(* Logix 5000 AddOnInstructionDefinition export SPEL_BaseSet; software revision 30.01 *)

ADD_ON_INSTRUCTION SPEL_ExecCmd   (* revision 1.2 *)
// Executes a command in the robot controller.  Normally this is called by higher level AOIs.
VAR_INPUT
   Start : BOOL; {required}
   MaxTime : DINT := 3000; {required}
END_VAR
VAR_OUTPUT
   InCycle : BOOL; {access Read Only, visible}
   Done : BOOL; {access Read Only, visible}
   Error : BOOL; {access Read Only, visible}
END_VAR
VAR_IN_OUT
   ExtInputs : AB:ETHERNET_MODULE_INT_128Bytes:I:0; {required}
        .DATA[0].0   // ExtCmdGet
        .DATA[0].1   // ExtRespSet
        .DATA[0].2   // ExtCmdResult
        .DATA[0].3   // ExtError
   ExtOutputs : AB:ETHERNET_MODULE_INT_128Bytes:O:0; {required}
        .DATA[0].0   // ExtCmdSet
        .DATA[0].1   // ExtRespGet
        .DATA[0].2   // ExtCmdReset
END_VAR
VAR_INPUT
   Cmd : INT; {required}
   CmdParam1 : INT; {required}
   CmdParam2 : INT; {required}
   CmdParam3 : INT; {required}
   CmdParam4 : INT; {required}
   CmdParam5 : INT; {required}
   CmdParam6 : INT; {required}
   CmdParam7 : INT; {required}
END_VAR
VAR_OUTPUT
   CmdEcho : INT; {access Read Only, visible}
   Resp1 : INT; {access Read Only, visible}
   Resp2 : INT; {access Read Only, visible}
   Resp3 : INT; {access Read Only, visible}
   Resp4 : INT; {access Read Only, visible}
   Resp5 : INT; {access Read Only, visible}
   Resp6 : INT; {access Read Only, visible}
   Resp7 : INT; {access Read Only, visible}
   ErrCode1 : INT; {access Read Only, visible}
   ErrCode2 : INT; {access Read Only, visible}
END_VAR
VAR
   ExtReset : BOOL; {access None}
   ExtError : BOOL; {access None}
   ExtCmdSet : BOOL; {access None}   // Cmd Ready
   ExtCmdGet : BOOL; {access None}   // Cmd Received
   CmdXferDone : BOOL; {access None}
   ExtRespSet : BOOL; {access None}   // Resp Ready
   RespXferDone : BOOL; {access None}
   ExtCmdResult : BOOL; {access None}   // Normal or Error?
   TmrCmdDataRdy : TIMER := (PRE := 5); {access None}
   OneShotDoneOff : BOOL; {access None}
   OneShotStart : BOOL; {access None}
   StartInit : BOOL; {access None}
   OneShotStartError : BOOL; {access None}
   TmrCycle : TIMER := (PRE := 5000); {access None}
   OneshotTmrPreset : BOOL; {access None}
   TmrCmdSet : TIMER := (PRE := 20); {access None}
   OnShotCmdDataXfer : BOOL; {access None}
   OneShotRespDataXfer : BOOL; {access None}
   OneShotDataRdy : BOOL; {access None}
   OtherCmdInCycle : BOOL; {access None}
   s : BOOL; {access None}
   OneShotUnsetCmdIncycle : BOOL; {access None}
   OneShotSetCmdIncycle : BOOL; {access None}
   OneShotSetOtherCmdInCycleError : BOOL; {access None}
   OneShotSetBit : BOOL; {access None}
   MaxTimeError : BOOL; {access None}
END_VAR

ROUTINE Logic   (* ladder *)
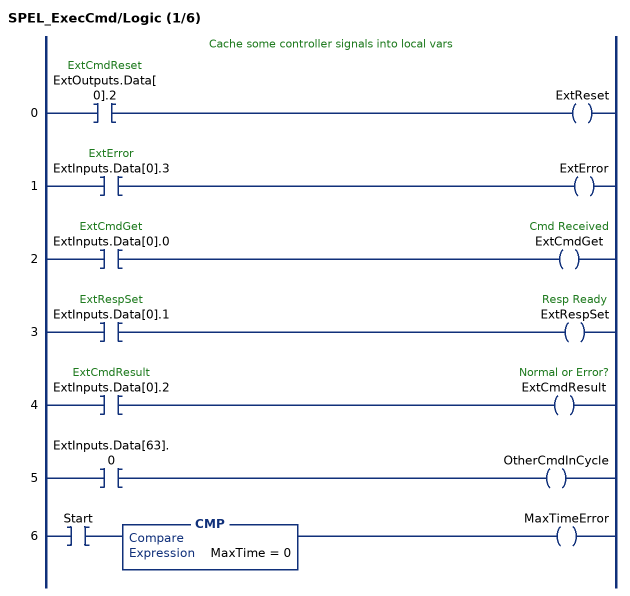
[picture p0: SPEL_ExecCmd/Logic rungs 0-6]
   // Cache some controller signals into local vars
   0: XIC(ExtOutputs.Data[0].2)OTE(ExtReset);
   1: XIC(ExtInputs.Data[0].3)OTE(ExtError);
   2: XIC(ExtInputs.Data[0].0)OTE(ExtCmdGet);
   3: XIC(ExtInputs.Data[0].1)OTE(ExtRespSet);
   4: XIC(ExtInputs.Data[0].2)OTE(ExtCmdResult);
   5: XIC(ExtInputs.Data[63].0)OTE(OtherCmdInCycle);
   6: XIC(Start)CMP(MaxTime = 0)OTE(MaxTimeError);
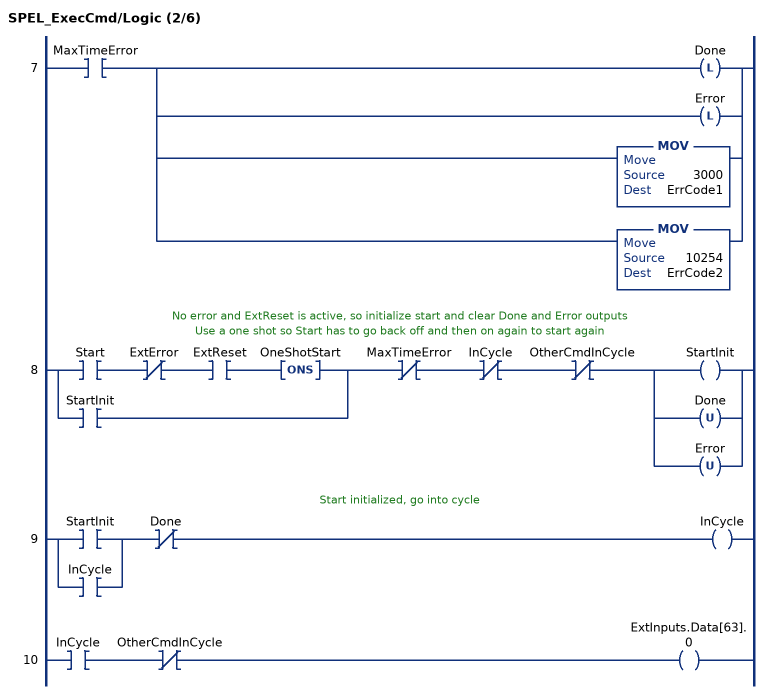
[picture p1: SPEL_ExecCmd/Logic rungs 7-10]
   7: XIC(MaxTimeError)[OTL(Done) ,OTL(Error) ,MOV(3000,ErrCode1) ,MOV(10254,ErrCode2) ];
   // No error and ExtReset is active, so initialize start and clear Done and Error outputs
   // Use a one shot so Start has to go back off and then on again to start again
   8: [XIC(Start) XIO(ExtError) XIC(ExtReset) ONS(OneShotStart) ,XIC(StartInit) ]XIO(MaxTimeError)XIO(InCycle)XIO(OtherCmdInCycle)[OTE(StartInit) ,OTU(Done) ,OTU(Error) ];
   // Start initialized, go into cycle
   9: [XIC(StartInit) ,XIC(InCycle) ]XIO(Done)OTE(InCycle);
   10: XIC(InCycle)XIO(OtherCmdInCycle)OTE(ExtInputs.Data[63].0);
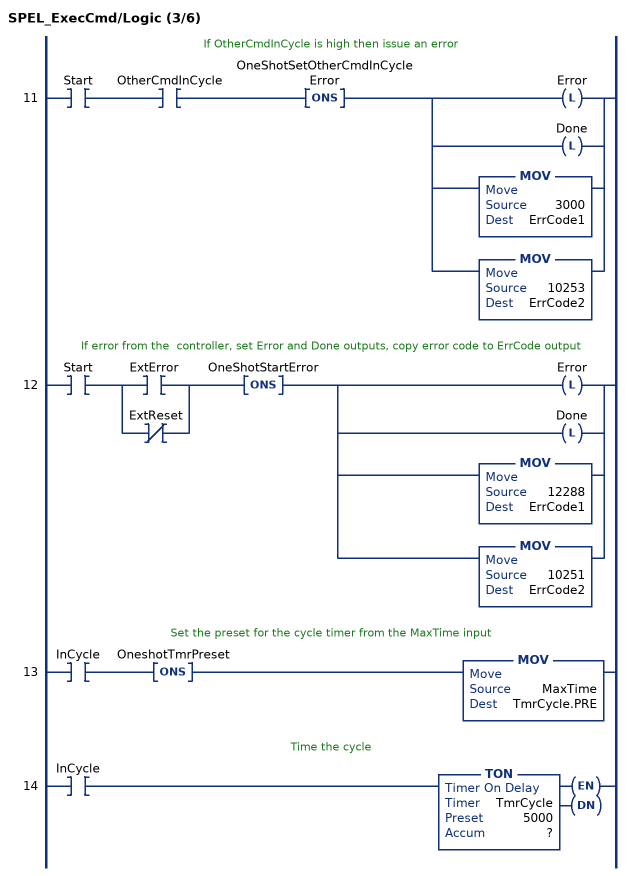
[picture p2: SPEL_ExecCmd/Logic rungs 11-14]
   // If OtherCmdInCycle is high then issue an error
   11: XIC(Start)XIC(OtherCmdInCycle)ONS(OneShotSetOtherCmdInCycleError)[OTL(Error) ,OTL(Done) ,MOV(3000,ErrCode1) ,MOV(10253,ErrCode2) ];
   // If error from the  controller, set Error and Done outputs, copy error code to ErrCode output
   12: XIC(Start)[XIC(ExtError) ,XIO(ExtReset) ]ONS(OneShotStartError)[OTL(Error) ,OTL(Done) ,MOV(12288,ErrCode1) ,MOV(10251,ErrCode2) ];
   // Set the preset for the cycle timer from the MaxTime input
   13: XIC(InCycle)ONS(OneshotTmrPreset)MOV(MaxTime,TmrCycle.PRE);
   // Time the cycle
   14: XIC(InCycle)TON(TmrCycle,?,?);
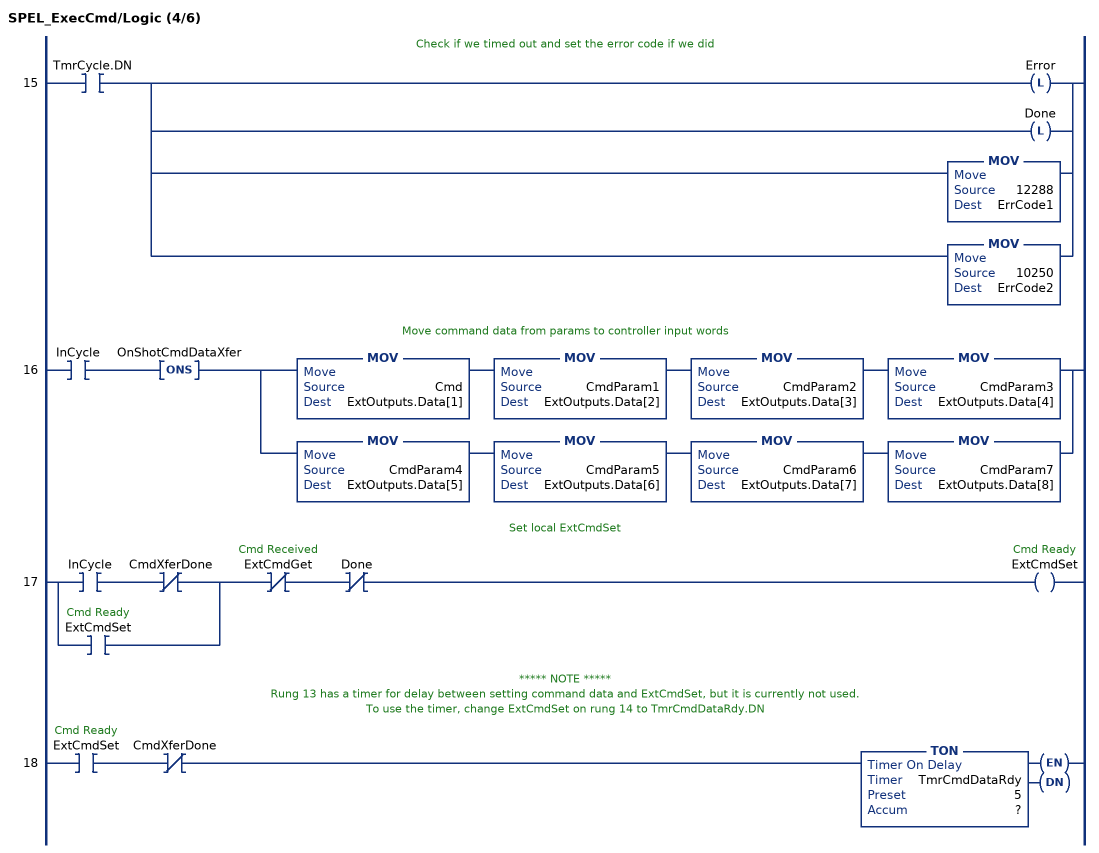
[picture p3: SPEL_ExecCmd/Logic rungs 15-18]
   // Check if we timed out and set the error code if we did
   15: XIC(TmrCycle.DN)[OTL(Error) ,OTL(Done) ,MOV(12288,ErrCode1) ,MOV(10250,ErrCode2) ];
   // Move command data from params to controller input words
   16: XIC(InCycle)ONS(OnShotCmdDataXfer)[MOV(Cmd,ExtOutputs.Data[1]) MOV(CmdParam1,ExtOutputs.Data[2]) MOV(CmdParam2,ExtOutputs.Data[3]) MOV(CmdParam3,ExtOutputs.Data[4]) ,MOV(CmdParam4,ExtOutputs.Data[5]) MOV(CmdParam5,ExtOutputs.Data[6]) MOV(CmdParam6,ExtOutputs.Data[7]) MOV(CmdParam7,ExtOutputs.Data[8]) ];
   // Set local ExtCmdSet
   17: [XIC(InCycle) XIO(CmdXferDone) ,XIC(ExtCmdSet) ]XIO(ExtCmdGet)XIO(Done)OTE(ExtCmdSet);
   // ***** NOTE *****
   // Rung 13 has a timer for delay between setting command data and ExtCmdSet, but it is currently not used.
   // To use the timer, change ExtCmdSet on rung 14 to TmrCmdDataRdy.DN
   18: XIC(ExtCmdSet)XIO(CmdXferDone)TON(TmrCmdDataRdy,?,?);
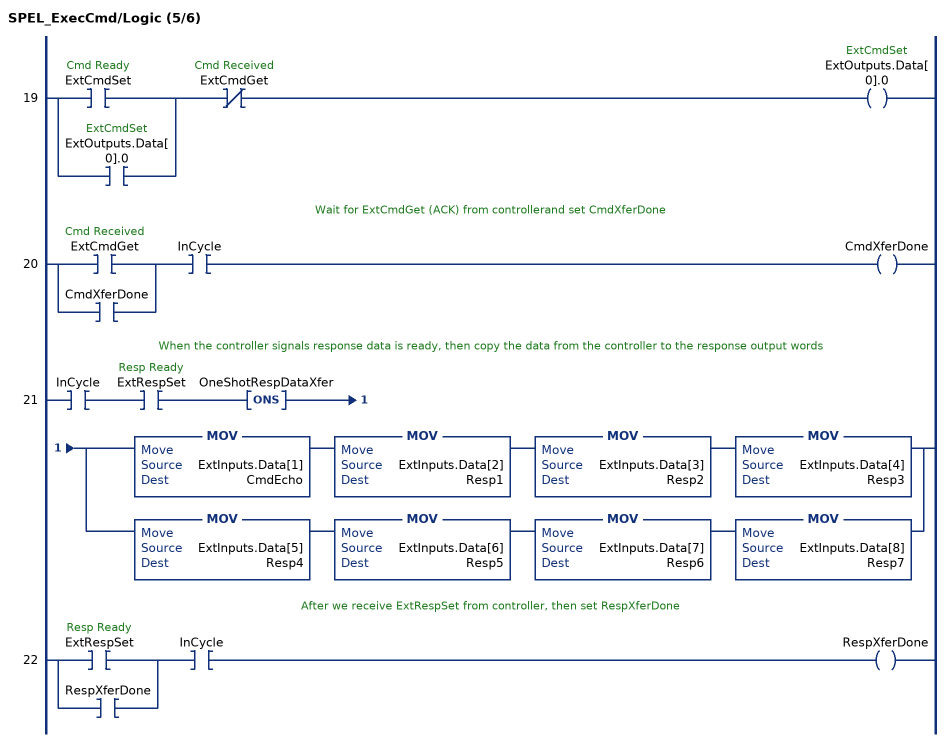
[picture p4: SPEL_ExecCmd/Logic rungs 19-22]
   19: [XIC(ExtCmdSet) ,XIC(ExtOutputs.Data[0].0) ]XIO(ExtCmdGet)OTE(ExtOutputs.Data[0].0);
   // Wait for ExtCmdGet (ACK) from controllerand set CmdXferDone
   20: [XIC(ExtCmdGet) ,XIC(CmdXferDone) ]XIC(InCycle)OTE(CmdXferDone);
   // When the controller signals response data is ready, then copy the data from the controller to the response output words
   21: XIC(InCycle)XIC(ExtRespSet)ONS(OneShotRespDataXfer)[MOV(ExtInputs.Data[1],CmdEcho) MOV(ExtInputs.Data[2],Resp1) MOV(ExtInputs.Data[3],Resp2) MOV(ExtInputs.Data[4],Resp3) ,MOV(ExtInputs.Data[5],Resp4) MOV(ExtInputs.Data[6],Resp5) MOV(ExtInputs.Data[7],Resp6) MOV(ExtInputs.Data[8],Resp7) ];
   // After we receive ExtRespSet from controller, then set RespXferDone
   22: [XIC(ExtRespSet) ,XIC(RespXferDone) ]XIC(InCycle)OTE(RespXferDone);
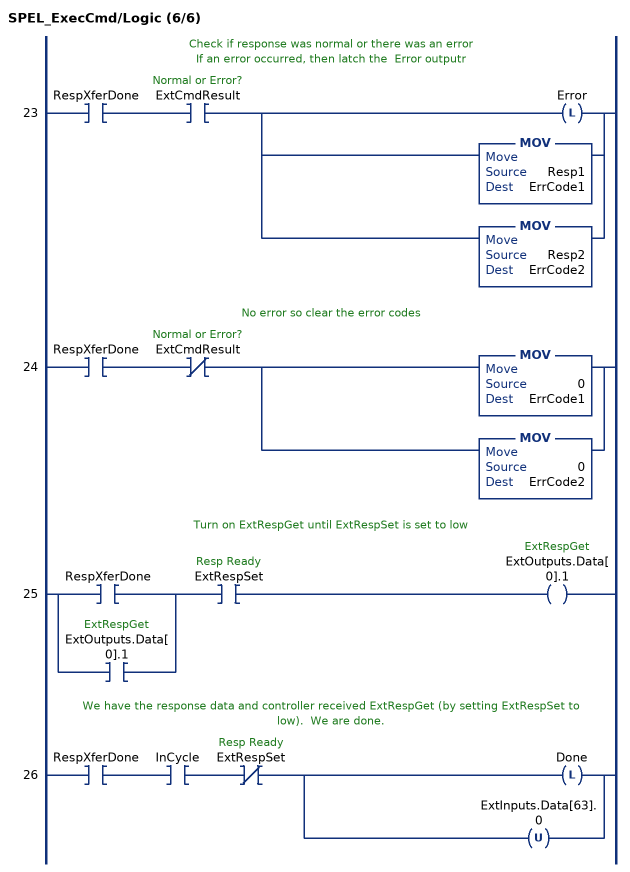
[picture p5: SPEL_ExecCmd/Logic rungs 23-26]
   // Check if response was normal or there was an error
   // If an error occurred, then latch the  Error outputr
   23: XIC(RespXferDone)XIC(ExtCmdResult)[OTL(Error) ,MOV(Resp1,ErrCode1) ,MOV(Resp2,ErrCode2) ];
   // No error so clear the error codes
   24: XIC(RespXferDone)XIO(ExtCmdResult)[MOV(0,ErrCode1) ,MOV(0,ErrCode2) ];
   // Turn on ExtRespGet until ExtRespSet is set to low
   25: [XIC(RespXferDone) ,XIC(ExtOutputs.Data[0].1) ]XIC(ExtRespSet)OTE(ExtOutputs.Data[0].1);
   // We have the response data and controller received ExtRespGet (by setting ExtRespSet to low).  We are done.
   26: XIC(RespXferDone)XIC(InCycle)XIO(ExtRespSet)[OTL(Done) ,OTU(ExtInputs.Data[63].0) ];
END_ROUTINE
END_ADD_ON_INSTRUCTION

ADD_ON_INSTRUCTION SPEL_BaseSet   (* revision 1.2, vendor SEIKO EPSON CORP. *)
// Sets the base coordinate system.
VAR_OUTPUT
   InCycle : BOOL; {access Read Only, visible}
   Done : BOOL; {access Read Only, visible}
END_VAR
VAR_INPUT
   Start : BOOL; {required}
END_VAR
VAR_OUTPUT
   Error : BOOL; {access Read Only, visible}
END_VAR
VAR_INPUT
   NumAxes : INT; {required}
   BaseX : REAL; {required}
   BaseY : REAL; {required}
   BaseZ : REAL; {required}
   BaseU : REAL; {required}
   BaseV : REAL; {required}
   BaseW : REAL; {required}
END_VAR
VAR_IN_OUT
   ExtInputs : AB:ETHERNET_MODULE_INT_128Bytes:I:0; {required}
   ExtOutputs : AB:ETHERNET_MODULE_INT_128Bytes:O:0; {required}
END_VAR
VAR_OUTPUT
   ErrCode1 : INT; {access Read Only, visible}
   ErrCode2 : INT; {access Read Only, visible}
END_VAR
VAR
   Valuex1000 : DINT; {access None}
   Value_INTS : INT[2]; {access None}
   StartInit : BOOL[32]; {access None}
   OneShotStart : BOOL[32]; {access None}
   ExecBaseSetX : SPEL_ExecCmd := (MaxTime := 3000); {access None}
   ExecBaseSetW : SPEL_ExecCmd := (MaxTime := 3000); {access None}
   ExecBaseSetV : SPEL_ExecCmd := (MaxTime := 3000); {access None}
   ExecBaseSetU : SPEL_ExecCmd := (MaxTime := 3000); {access None}
   ExecBaseSetZ : SPEL_ExecCmd := (MaxTime := 3000); {access None}
   ExecBaseSetY : SPEL_ExecCmd := (MaxTime := 3000); {access None}
   X6 : BOOL; {access None}
   ExecTimeout : DINT; {access None}
END_VAR

ROUTINE Logic   (* ladder *)
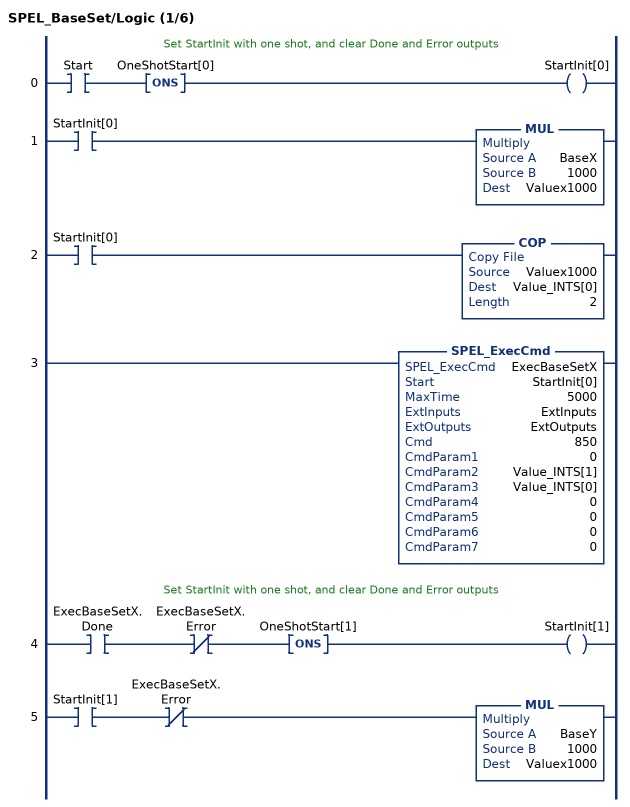
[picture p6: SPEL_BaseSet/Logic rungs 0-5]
   // Set StartInit with one shot, and clear Done and Error outputs
   0: XIC(Start)ONS(OneShotStart[0])OTE(StartInit[0]);
   1: XIC(StartInit[0])MUL(BaseX,1000,Valuex1000);
   2: XIC(StartInit[0])COP(Valuex1000,Value_INTS[0],2);
   3: SPEL_ExecCmd(ExecBaseSetX,StartInit[0],5000,ExtInputs,ExtOutputs,850,0,Value_INTS[1],Value_INTS[0],0,0,0,0);
   // Set StartInit with one shot, and clear Done and Error outputs
   4: XIC(ExecBaseSetX.Done)XIO(ExecBaseSetX.Error)ONS(OneShotStart[1])OTE(StartInit[1]);
   5: XIC(StartInit[1])XIO(ExecBaseSetX.Error)MUL(BaseY,1000,Valuex1000);
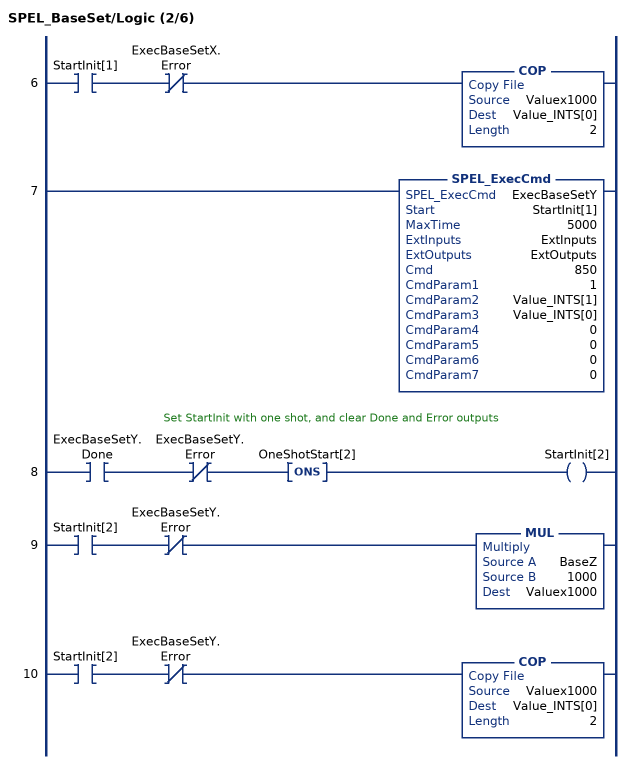
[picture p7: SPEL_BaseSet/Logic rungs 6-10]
   6: XIC(StartInit[1])XIO(ExecBaseSetX.Error)COP(Valuex1000,Value_INTS[0],2);
   7: SPEL_ExecCmd(ExecBaseSetY,StartInit[1],5000,ExtInputs,ExtOutputs,850,1,Value_INTS[1],Value_INTS[0],0,0,0,0);
   // Set StartInit with one shot, and clear Done and Error outputs
   8: XIC(ExecBaseSetY.Done)XIO(ExecBaseSetY.Error)ONS(OneShotStart[2])OTE(StartInit[2]);
   9: XIC(StartInit[2])XIO(ExecBaseSetY.Error)MUL(BaseZ,1000,Valuex1000);
   10: XIC(StartInit[2])XIO(ExecBaseSetY.Error)COP(Valuex1000,Value_INTS[0],2);
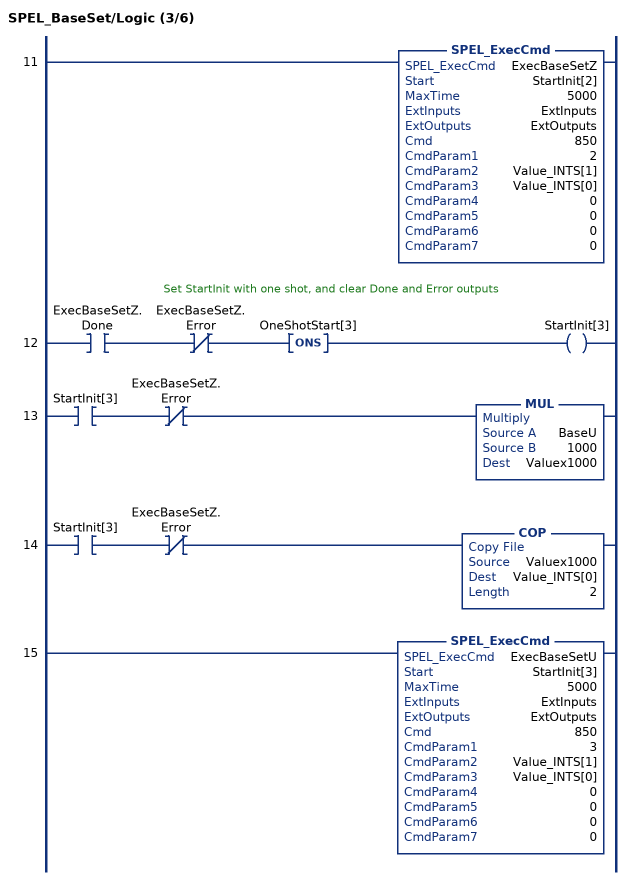
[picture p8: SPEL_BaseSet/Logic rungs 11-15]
   11: SPEL_ExecCmd(ExecBaseSetZ,StartInit[2],5000,ExtInputs,ExtOutputs,850,2,Value_INTS[1],Value_INTS[0],0,0,0,0);
   // Set StartInit with one shot, and clear Done and Error outputs
   12: XIC(ExecBaseSetZ.Done)XIO(ExecBaseSetZ.Error)ONS(OneShotStart[3])OTE(StartInit[3]);
   13: XIC(StartInit[3])XIO(ExecBaseSetZ.Error)MUL(BaseU,1000,Valuex1000);
   14: XIC(StartInit[3])XIO(ExecBaseSetZ.Error)COP(Valuex1000,Value_INTS[0],2);
   15: SPEL_ExecCmd(ExecBaseSetU,StartInit[3],5000,ExtInputs,ExtOutputs,850,3,Value_INTS[1],Value_INTS[0],0,0,0,0);
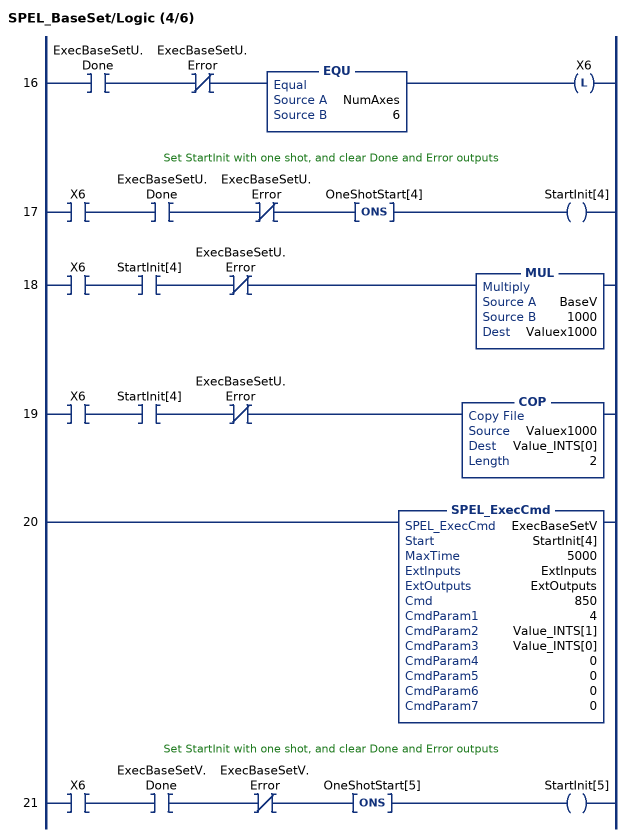
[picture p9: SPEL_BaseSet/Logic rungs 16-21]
   16: XIC(ExecBaseSetU.Done)XIO(ExecBaseSetU.Error)EQU(NumAxes,6)OTL(X6);
   // Set StartInit with one shot, and clear Done and Error outputs
   17: XIC(X6)XIC(ExecBaseSetU.Done)XIO(ExecBaseSetU.Error)ONS(OneShotStart[4])OTE(StartInit[4]);
   18: XIC(X6)XIC(StartInit[4])XIO(ExecBaseSetU.Error)MUL(BaseV,1000,Valuex1000);
   19: XIC(X6)XIC(StartInit[4])XIO(ExecBaseSetU.Error)COP(Valuex1000,Value_INTS[0],2);
   20: SPEL_ExecCmd(ExecBaseSetV,StartInit[4],5000,ExtInputs,ExtOutputs,850,4,Value_INTS[1],Value_INTS[0],0,0,0,0);
   // Set StartInit with one shot, and clear Done and Error outputs
   21: XIC(X6)XIC(ExecBaseSetV.Done)XIO(ExecBaseSetV.Error)ONS(OneShotStart[5])OTE(StartInit[5]);
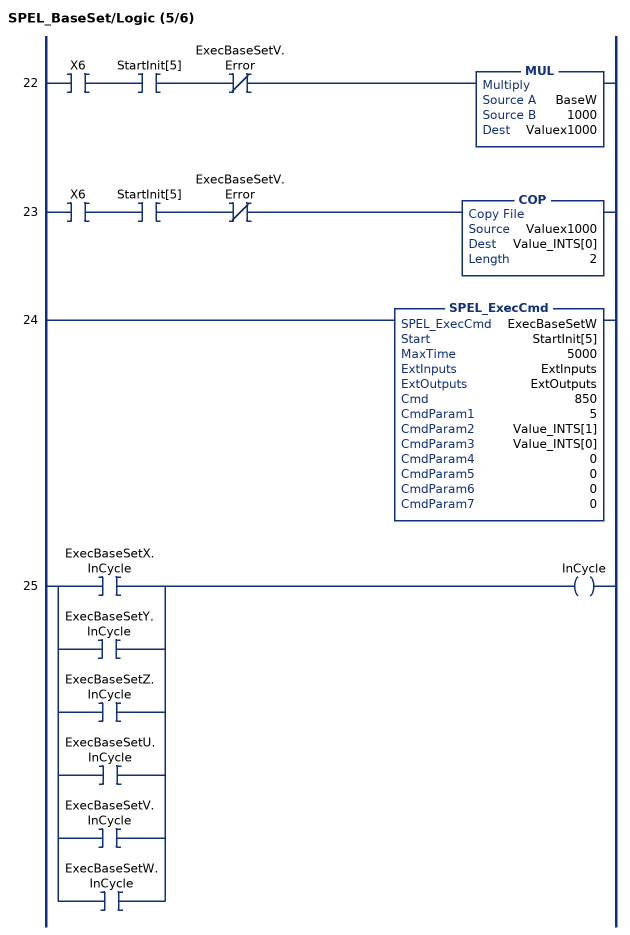
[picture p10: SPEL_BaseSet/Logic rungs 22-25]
   22: XIC(X6)XIC(StartInit[5])XIO(ExecBaseSetV.Error)MUL(BaseW,1000,Valuex1000);
   23: XIC(X6)XIC(StartInit[5])XIO(ExecBaseSetV.Error)COP(Valuex1000,Value_INTS[0],2);
   24: SPEL_ExecCmd(ExecBaseSetW,StartInit[5],5000,ExtInputs,ExtOutputs,850,5,Value_INTS[1],Value_INTS[0],0,0,0,0);
   25: [XIC(ExecBaseSetX.InCycle) ,XIC(ExecBaseSetY.InCycle) ,XIC(ExecBaseSetZ.InCycle) ,XIC(ExecBaseSetU.InCycle) ,XIC(ExecBaseSetV.InCycle) ,XIC(ExecBaseSetW.InCycle) ]OTE(InCycle);
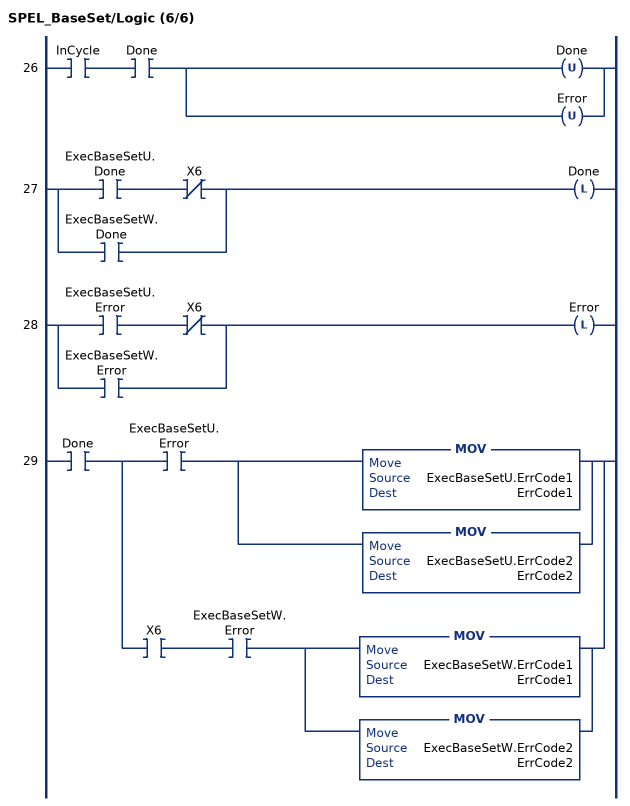
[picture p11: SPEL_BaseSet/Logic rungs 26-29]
   26: XIC(InCycle)XIC(Done)[OTU(Done) ,OTU(Error) ];
   27: [XIC(ExecBaseSetU.Done) XIO(X6) ,XIC(ExecBaseSetW.Done) ]OTL(Done);
   28: [XIC(ExecBaseSetU.Error) XIO(X6) ,XIC(ExecBaseSetW.Error) ]OTL(Error);
   29: XIC(Done)[XIC(ExecBaseSetU.Error) [MOV(ExecBaseSetU.ErrCode1,ErrCode1) ,MOV(ExecBaseSetU.ErrCode2,ErrCode2) ] ,XIC(X6) XIC(ExecBaseSetW.Error) [MOV(ExecBaseSetW.ErrCode1,ErrCode1) ,MOV(ExecBaseSetW.ErrCode2,ErrCode2) ] ];
END_ROUTINE
END_ADD_ON_INSTRUCTION
